FUNCTION FC 50 : VOID
TITLE =
VERSION : 0.1

BEGIN
NETWORK
TITLE =Call alarm function press

NETWORK
TITLE =Call partcontrol function press

      CALL FC    53 ;
      NOP   0;
NETWORK
TITLE =Call auto function press

      CALL FC    55 ;

      NOP   0;
NETWORK
TITLE =Call valve function press

      CALL FC    56 ;

      NOP   0;
NETWORK
TITLE =Call output function press

      CALL FC    57 ;

      NOP   0;
END_FUNCTION

